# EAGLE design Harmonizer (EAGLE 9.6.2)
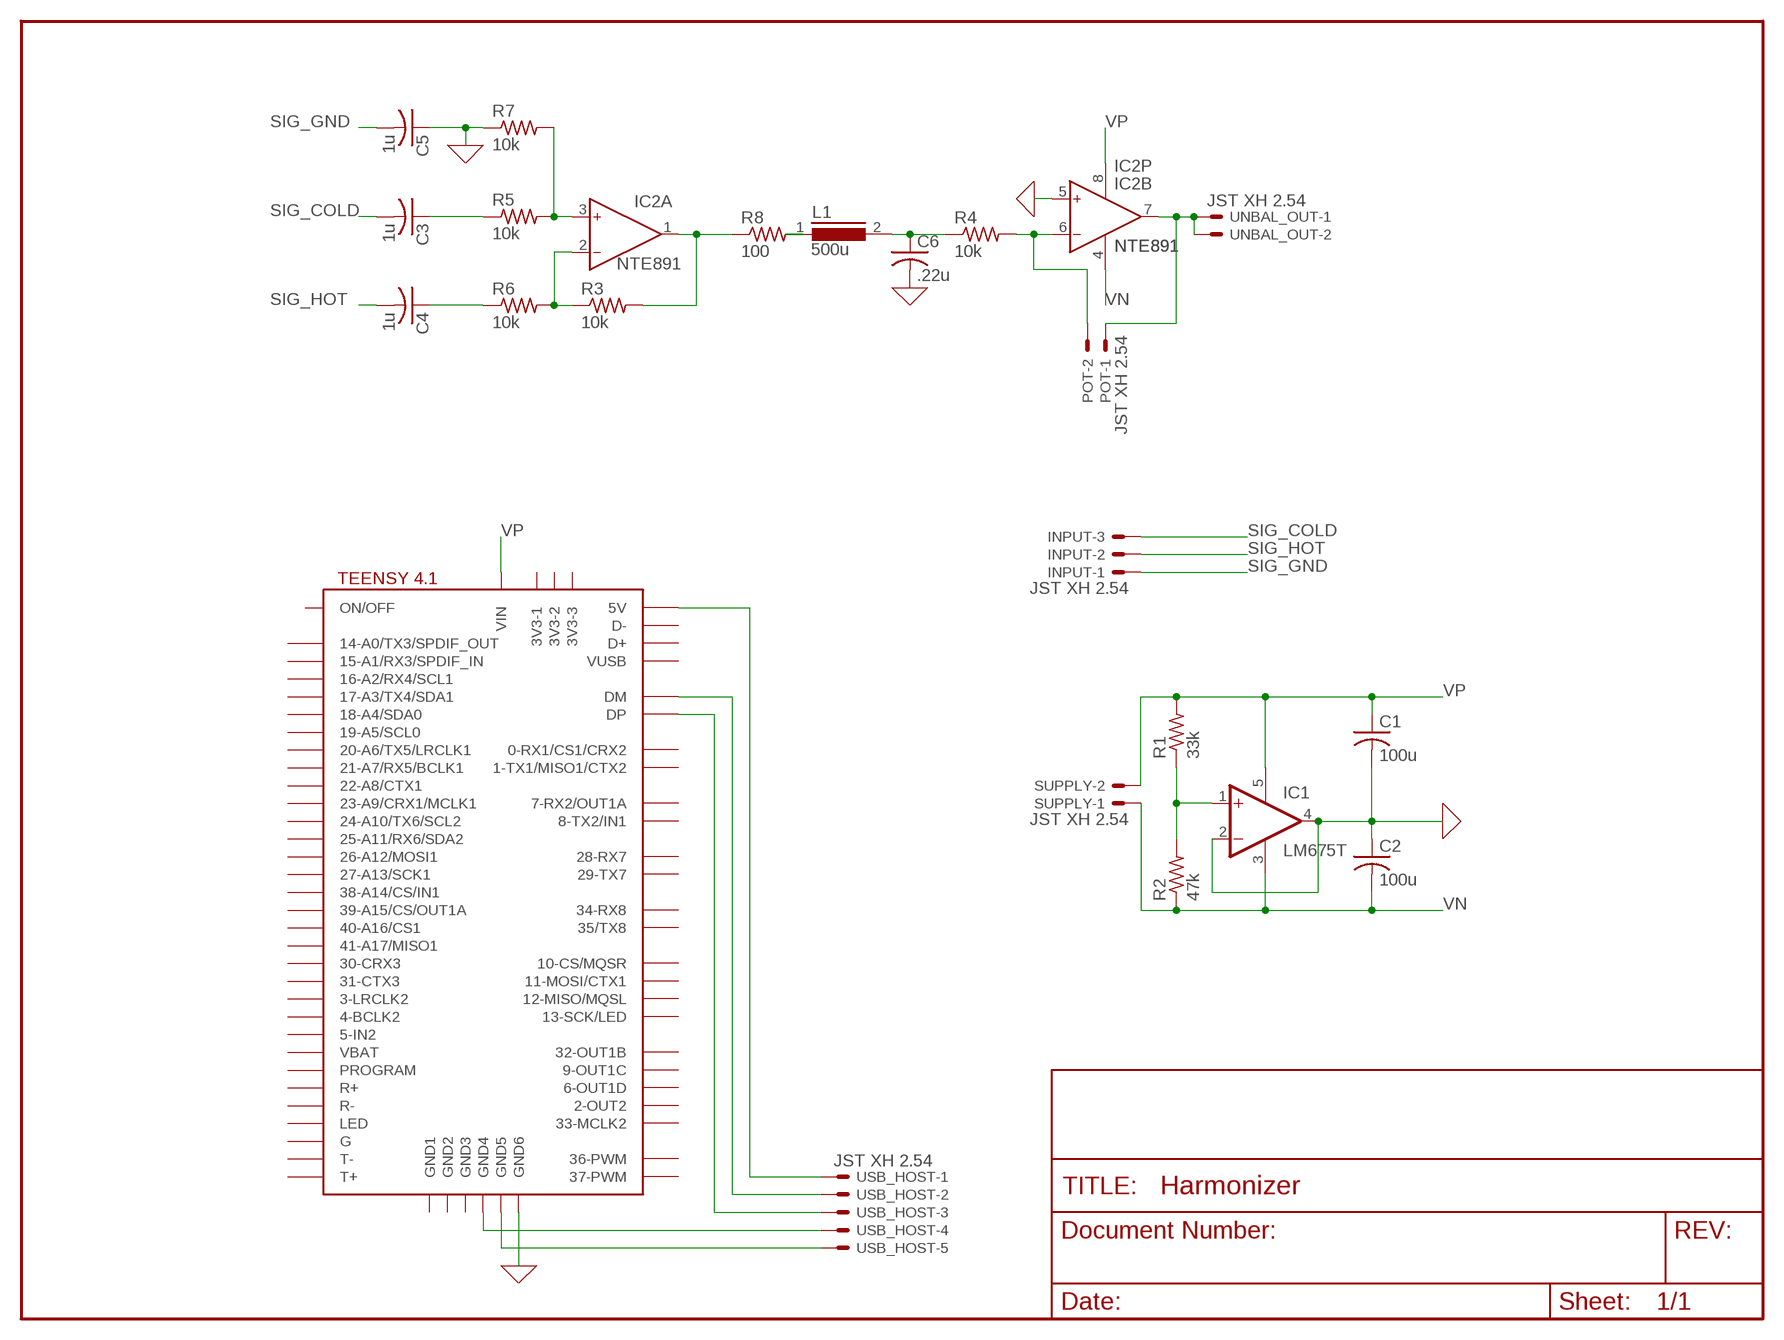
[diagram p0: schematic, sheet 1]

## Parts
C1  100u  C-USC025-050X050-BANTAM  [C025-050X050-BANTAM]
C2  100u  C-USC025-050X050-BANTAM  [C025-050X050-BANTAM]
C3  1u  C-USC025-050X050-BANTAM  [C025-050X050-BANTAM]
C4  1u  C-USC025-050X050-BANTAM  [C025-050X050-BANTAM]
C5  1u  C-USC025-050X050-BANTAM  [C025-050X050-BANTAM]
C6  .22u  C-USC025-050X050-BANTAM  [C025-050X050-BANTAM]
IC1  LM675T  [CB367]
IC2  NTE891  AD822N  [DIL08]
INPUT  JST XH 2.54  22-23-2031  [22-23-2031]
L1  500u  B82134  [SUKW4-32]
POT  JST XH 2.54  22-23-2021  [22-23-2021]
R1  33k  R-US_0207/10-BANTAM  [0207/10-BANTAM]
R2  47k  R-US_0207/10-BANTAM  [0207/10-BANTAM]
R3  10k  R-US_0207/10-BANTAM  [0207/10-BANTAM]
R4  10k  R-US_0207/10-BANTAM  [0207/10-BANTAM]
R5  10k  R-US_0207/10-BANTAM  [0207/10-BANTAM]
R6  10k  R-US_0207/10-BANTAM  [0207/10-BANTAM]
R7  10k  R-US_0207/10-BANTAM  [0207/10-BANTAM]
R8  100  R-US_0207/10-BANTAM  [0207/10-BANTAM]
SUPPLY  JST XH 2.54  22-27-2021-02  [6410-02]
U$1  TEENSY41  [TEENSY41]
UNBAL_OUT  JST XH 2.54  22-27-2021-02  [6410-02]
USB_HOST  JST XH 2.54  22-27-2051-05  [6410-05]

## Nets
0: C1.2 C2.1 C5.1 C6.2 IC1.2(-IN) IC1.4(OUT) IC2.5(B:IN+) R7.1 U$1.GND6 ; supply symbol labelled GND
N$1: IC2.1(A:OUT) R3.2 R8.1
N$2: IC2.6(B:IN-) POT.2 R4.2
N$3: C6.1 L1.2 R4.1
N$4: IC2.2(A:IN-) R3.1 R6.2
N$5: IC2.3(A:IN+) R5.2 R7.2
N$6: L1.1 R8.2
N$7: IC1.1(+IN) R1.1 R2.2
N$8: C3.1 R5.1
N$9: C4.1 R6.1
N$10: U$1.GND5 USB_HOST.5
N$11: U$1.GND4 USB_HOST.4
N$12: U$1.DP USB_HOST.3
N$13: U$1.DM USB_HOST.2
N$14: U$1.+5V(5V) USB_HOST.1
SIG_COLD: C3.2 INPUT.3
SIG_GND: C5.2 INPUT.1
SIG_HOT: C4.2 INPUT.2
UNBAL_OUT: IC2.7(B:OUT) POT.1 UNBAL_OUT.1 UNBAL_OUT.2
VN: C2.2 IC1.3(V-) IC2.4(P:V-) R2.1 SUPPLY.1
VP: C1.1 IC1.5(V+) IC2.8(P:V+) R1.2 SUPPLY.2 U$1.VIN
Unconnected: U$1.0-RX1/CS1/CRX2 U$1.1-TX1/MISO1/CTX2 U$1.2-OUT2 U$1.3-LRCLK2 U$1.3V3-1 U$1.3V3-2 U$1.3V3-3 U$1.4-BCLK2 U$1.5-IN2 U$1.6-OUT1D U$1.7-RX2/OUT1A U$1.8-TX2/IN2(8-TX2/IN1) U$1.9-OUT1C U$1.10-CS\MQSR(10-CS/MQSR) U$1.11-MOSI/CTX1 U$1.12-MISO/MQSL U$1.13-SCK/LED U$1.14-A0/TX3/SPDIF_OUT U$1.15-A1/RX3/SPDIF_IN U$1.16-A2/RX4/SCL1 U$1.17-A3/TX4/SDA1 U$1.18-A4/SDA0 U$1.19-A5/SCL0 U$1.20-A6/TX5/LRCLK1 U$1.21-A7/RX5/BCLK1 U$1.22-A8/CTX1 U$1.23-A9/CRX1/MCLK1 U$1.24-A10/TX6/SCL2 U$1.25-A11/RX6/SDA2 U$1.26-A12/MOSI1 U$1.27-A13/SCK1 U$1.28-RX7 U$1.29-TX7 U$1.30-CRX3 U$1.31-CTX3 U$1.32-OUT1B U$1.33-MCLK2 U$1.34-RX8 U$1.35-TX8(35/TX8) U$1.36-PWM U$1.37-PWM U$1.38-A14/CS/IN1 U$1.39-A15/CS/OUT1A U$1.40-A16/CS1 U$1.41-A17/MISO1 U$1.D+ U$1.D- U$1.G U$1.GND1 U$1.GND2 U$1.GND3 U$1.LED U$1.ON/OFF U$1.PROGRAM U$1.R+ U$1.R- U$1.T+ U$1.T- U$1.VBAT U$1.VUSB

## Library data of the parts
C1-C6 = rcl-custom:C-US: CAPACITOR, American symbol
IC1 = linear:LM675T: Power OP AMP
IC2 = analog-devices:AD822: Single-Supply, Rail-to-Rail Low Power FET-Input Op Amp Source: http://www.analog.com/static/imported-files/data_sheets/AD822.pdf; OC_FARNELL: 1438581; OC_NEWARK: unknown
INPUT = con-molex:22-23-2031: .100" (2.54mm) Center Header - 3 Pin; MF: MOLEX; MPN: 22-23-2031; OC_FARNELL: 1462950; OC_NEWARK: 30C0862
L1 = inductors:B82134: INDUCTOR; SPICEPREFIX: L
POT = con-molex:22-23-2021: .100" (2.54mm) Center Header - 2 Pin; MF: MOLEX; MPN: 22-23-2021; OC_FARNELL: 1462926; OC_NEWARK: 25C3832
R1-R8 = rcl-custom:R-US_: RESISTOR, American symbol
SUPPLY UNBAL_OUT = con-molex:22-?-02: CONNECTOR; MF: MOLEX; OC_FARNELL: unknown; OC_NEWARK: unknown
U$1 = TeensyReducedPinout:TEENSY41
USB_HOST = con-molex:22-?-05: CONNECTOR wire to board 2.54 mm (.1 inch) pitch header; MF: MOLEX; OC_FARNELL: unknown; OC_NEWARK: unknown

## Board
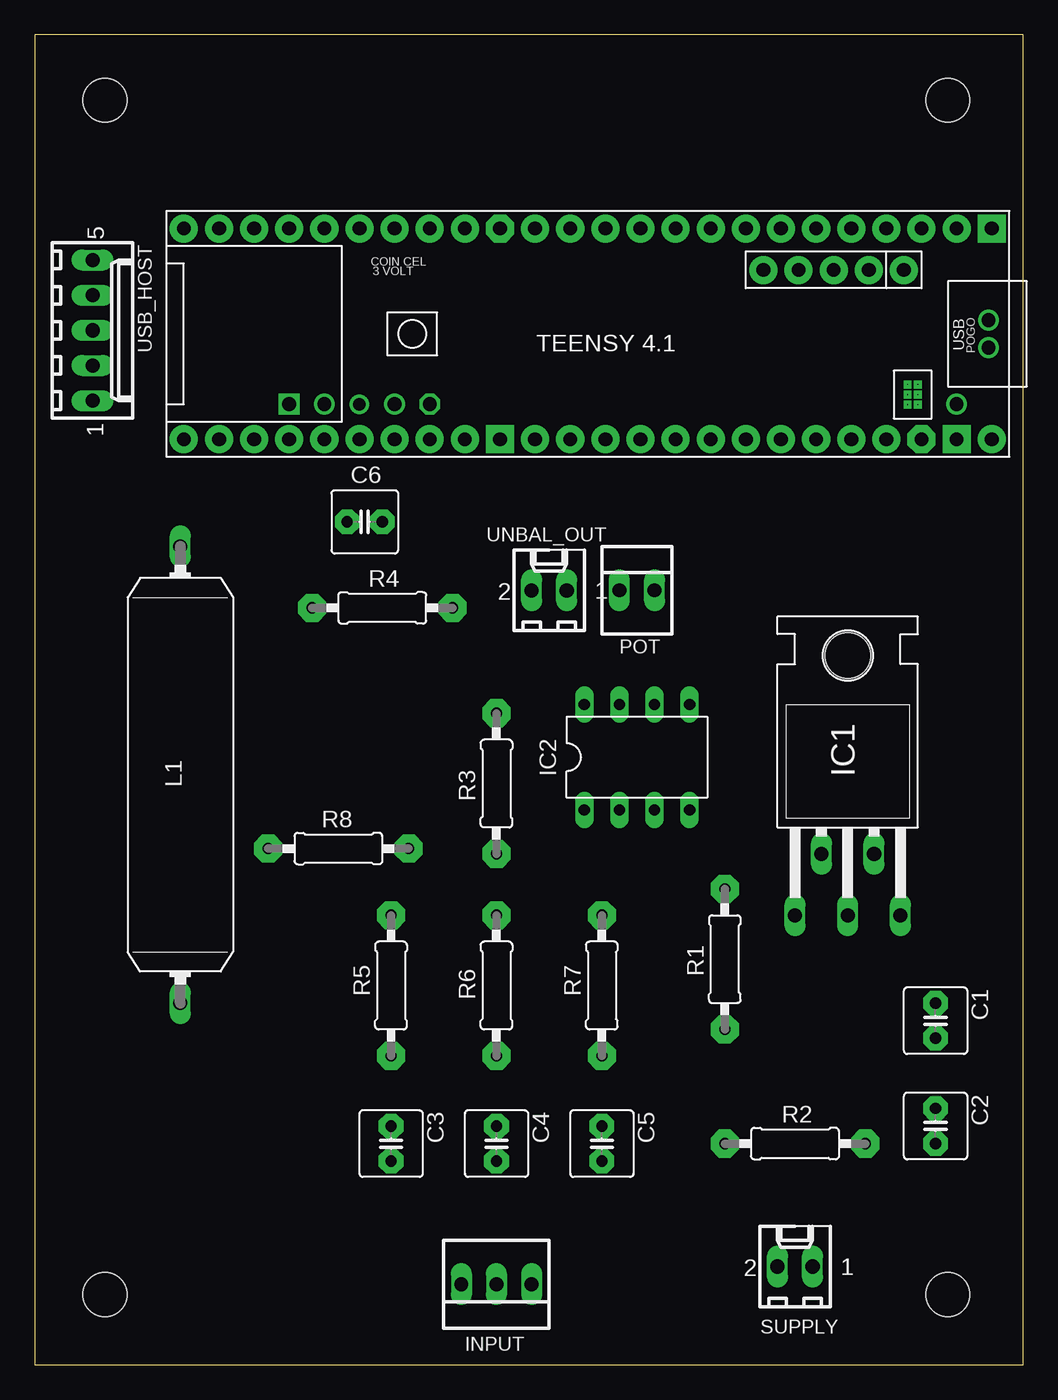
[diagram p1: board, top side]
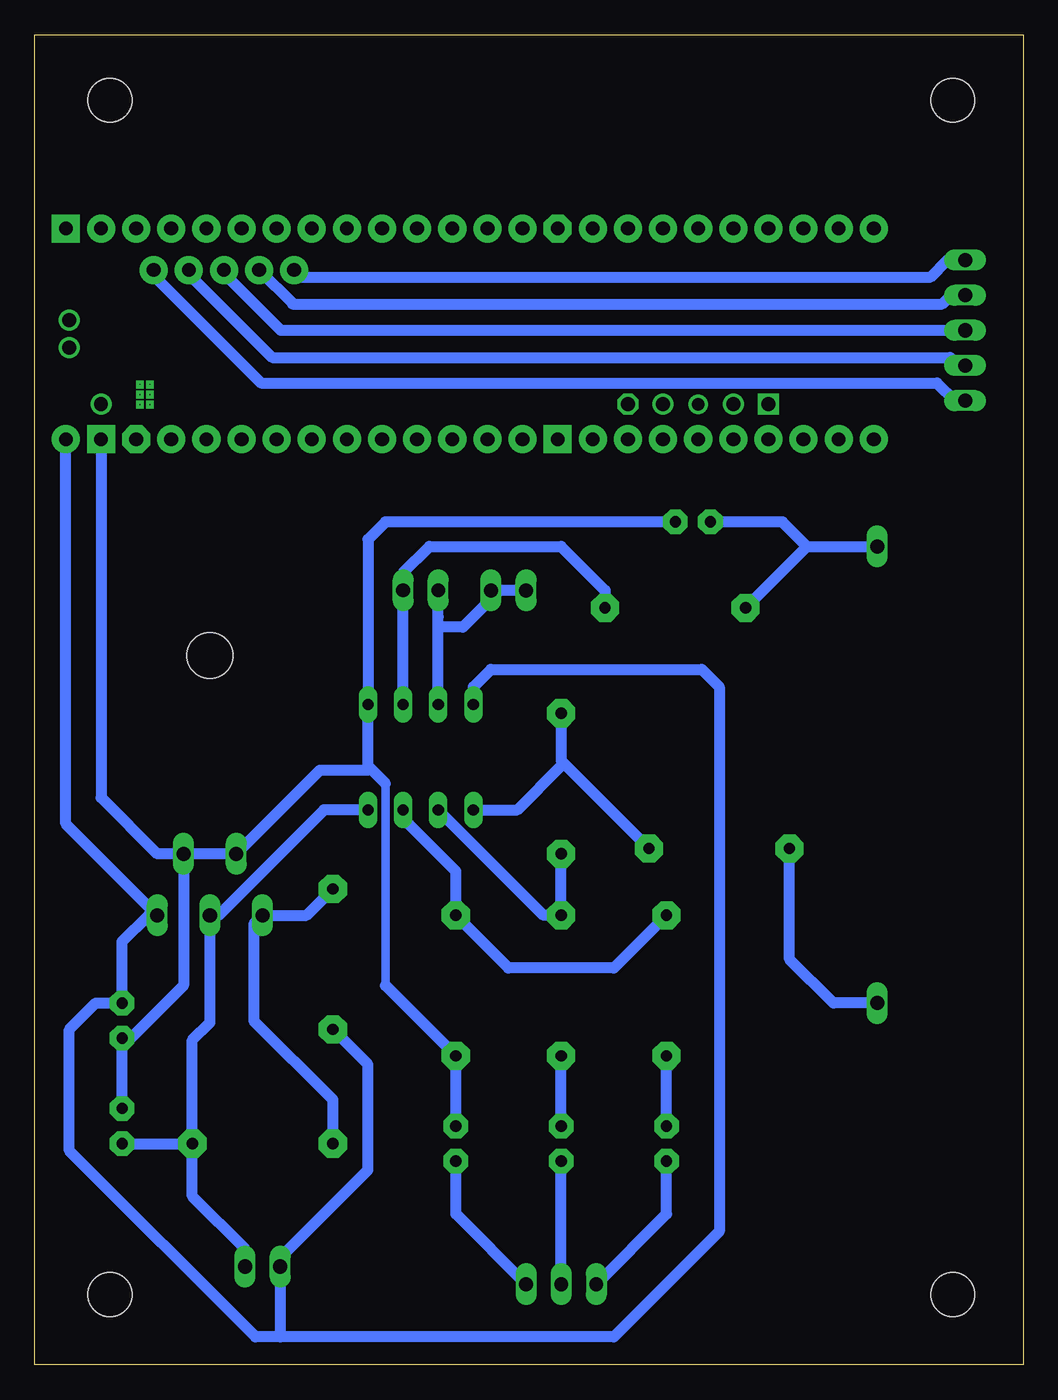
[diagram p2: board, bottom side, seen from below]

Size 71.48 x 96.19 mm. Coordinates in mm from the lower left corner, seen from the top.
Outline: 0,0 71.48,0 71.48,96.19 0,96.19 0,0
Copper layers (1*16): Top 0.035mm / dielectric 1.5mm / Bottom 0.035mm
Design rules "default": minimum track width 6mil, minimum drill 0.35mm, track to track 6mil, track to pad 6mil, pad to pad 6mil, via to via 6mil, smd to smd 6mil, copper to edge 40mil, drill to drill 6mil, minimum pad ring 10mil, minimum via ring 8mil, stop-mask expansion 4mil, vias tented up to drill 0mil, thermal gap 10mil
Holes 3.17 mm at 66.04,5.08 5.08,5.08 5.08,91.44 66.04,91.44

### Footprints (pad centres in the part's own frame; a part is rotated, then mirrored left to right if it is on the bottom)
C025-050X050-BANTAM = drill 0.813 pad 1.778 octagon: 1 -1.27,0; 2 1.27,0
CB367 = drill 1.016 long: 1 -3.81,-11.43; 2 -1.905,-6.985; 3 0,-11.43; 4 1.905,-6.985; 5 3.81,-11.43 | hole 3.302: 0,7.366
DIL08 = drill 0.813 long: 1 -3.81,-3.81; 2 -1.27,-3.81; 3 1.27,-3.81; 4 3.81,-3.81; 5 3.81,3.81; 6 1.27,3.81; 7 -1.27,3.81; 8 -3.81,3.81
22-23-2031 = drill 1 long: 1 -2.54,0; 2 0,0; 3 2.54,0
SUKW4-32 = drill 1.016 long: 1 -16.51,0; 2 16.51,0
22-23-2021 = drill 1 long: 1 -1.27,0; 2 1.27,0
0207/10-BANTAM = drill 0.813 pad 2.032 octagon: 1 -5.08,0; 2 5.08,0
6410-02 = drill 1.016 long: 1 1.27,0; 2 -1.27,0
TEENSY41 = drill 1 pad 2.032: 0-RX1/CS1/CRX2 -27.94,-7.62; 1-TX1/MISO1/CTX2 -25.4,-7.62; 2-OUT2 -22.86,-7.62; 3-LRCLK2 -20.32,-7.62; 4-BCLK2 -17.78,-7.62; 5-IN2 -15.24,-7.62; 6-OUT1D -12.7,-7.62; 7-RX2/OUT1A -10.16,-7.62; 8-TX2/IN2 -7.62,-7.62; 9-OUT1C -5.08,-7.62; 10-CS\MQSR -2.54,-7.62; 11-MOSI/CTX1 0,-7.62; 12-MISO/MQSL 2.54,-7.62; 13-SCK/LED 2.54,7.62; 14-A0/TX3/SPDIF_OUT 0,7.62; 15-A1/RX3/SPDIF_IN -2.54,7.62; 16-A2/RX4/SCL1 -5.08,7.62; 17-A3/TX4/SDA1 -7.62,7.62; 18-A4/SDA0 -10.16,7.62; 19-A5/SCL0 -12.7,7.62; 20-A6/TX5/LRCLK1 -15.24,7.62; 21-A7/RX5/BCLK1 -17.78,7.62; 22-A8/CTX1 -20.32,7.62; 23-A9/CRX1/MCLK1 -22.86,7.62; 24-A10/TX6/SCL2 7.62,-7.62; 25-A11/RX6/SDA2 10.16,-7.62; 26-A12/MOSI1 12.7,-7.62; 27-A13/SCK1 15.24,-7.62; 28-RX7 17.78,-7.62; 29-TX7 20.32,-7.62; 30-CRX3 22.86,-7.62; 31-CTX3 25.4,-7.62; 32-OUT1B 27.94,-7.62; 33-MCLK2 27.94,7.62; 34-RX8 25.4,7.62; 35-TX8 22.86,7.62; 36-PWM 20.32,7.62; 37-PWM 17.78,7.62; 38-A14/CS/IN1 15.24,7.62; 39-A15/CS/OUT1A 12.7,7.62; 40-A16/CS1 10.16,7.62; 41-A17/MISO1 7.62,7.62; +5V -24.13,-4.62; DM -21.59,-4.62; DP -19.05,-4.62; GND4 -16.51,-4.62; GND5 -13.97,-4.62; VIN -30.48,7.62 | drill 1 pad 2.032 octagon: 3V3-1 5.08,-7.62; 3V3-3 -25.4,7.62 | drill 1 pad 0.025: 3V3-2 17.78,5.08; PROGRAM 12.7,5.08 | drill 1: D+ -30.25,-1; D- -30.25,1; VUSB -27.94,5.08 | drill 0.051 pad 0.025 square: G -24.4,4.39; LED -25.13,4.39; R+ -25.13,5.12; R- -24.4,5.12; T+ -24.4,3.66; T- -25.13,3.66 | drill 1 pad 2.032 square: GND1 -30.48,-7.62; GND3 5.08,7.62; GND6 -27.94,7.62 | drill 0.9 pad 0.025: GND2 15.24,5.08 | drill 1 pad 0.025 octagon: ON/OFF 10.16,5.08 | drill 1 pad 0.025 square: VBAT 20.32,5.08
6410-05 = drill 1.016 long: 1 5.08,0; 2 2.54,0; 3 0,0; 4 -2.54,0; 5 -5.08,0

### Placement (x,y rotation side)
C1  65.15,24.89 270 top
C2  65.15,17.27 270 top
C3  25.78,16 270 top
C4  33.4,16 270 top
C5  41.02,16 270 top
C6  23.88,60.96 0 top
IC1  58.8,43.94 0 top
IC2  43.56,43.94 0 top
INPUT  33.4,5.84 180 top
L1  10.54,42.67 90 top
POT  43.56,56.01 0 top
R1  49.91,29.34 270 top
R2  54.99,16 180 top
R3  33.4,42.04 90 top
R4  25.15,54.74 0 top
R5  25.78,27.43 90 top
R6  33.4,27.43 90 top
R7  41.02,27.43 90 top
R8  21.97,37.34 180 top
SUPPLY  54.99,7.11 0 top
U$1  38.73,74.55 180 top
UNBAL_OUT  37.21,56.01 0 top
USB_HOST  4.19,74.8 270 top

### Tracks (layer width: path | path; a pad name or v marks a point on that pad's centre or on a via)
0
  Bottom 0.61: 46.1,42.04 46.1,27.43
  Bottom 0.813: C2.1 C1.2 64.52,23.62 60.71,27.43 IC1.4 | IC1.4 IC1.2 50.86,42.99 47.37,42.99 47.37,43.31 | C5.1 R7.1 46.1,27.43 | IC1.4 62.61,36.96 66.67,41.02 U$1.GND6 | 47.37,43.31 46.1,42.04 | C6.2 46.1,60.96 47.37,59.69 IC2.5 47.37,43.31
N$1
  Bottom 0.61: 33.4,43.31 R3.2
  Bottom 0.813: IC2.1 36.58,40.13 33.4,43.31 | R3.2 33.4,43.69 R8.1
N$2
  Bottom 0.61: POT.2 44.83,57.28
  Bottom 0.813: IC2.6 POT.2 | R4.2 30.23,56.01 33.4,59.18 42.93,59.18 44.83,57.28
N$3
  Bottom 0.813: 15.62,59.18 17.4,60.96 C6.1 | R4.1 15.62,59.18 | 15.62,59.18 L1.2
N$4
  Bottom 0.813: IC2.2 34.67,32.51 R6.2 R3.1
N$5
  Bottom 0.61: 44.83,39.5 IC2.3
  Bottom 0.813: R5.2 29.59,28.7 37.21,28.7 R7.2 41.02,35.69 44.83,39.5
N$6
  Bottom 0.813: L1.1 13.72,26.16 16.89,29.34 R8.2
N$7
  Bottom 0.813: R2.2 49.91,19.18 55.63,24.89 55.63,31.88 IC1.1 51.82,32.51 R1.1
N$8
  Bottom 0.813: C3.1 R5.1
N$9
  Bottom 0.813: C4.1 R6.1
N$10
  Bottom 0.813: U$1.GND5 52.2,78.66 6.68,78.66 5.46,79.88 USB_HOST.5
N$11
  Bottom 0.813: U$1.GND4 52.83,76.76 52.83,76.71 5.84,76.71 5.21,77.34 USB_HOST.4
N$12
  Bottom 0.406: U$1.DP 57.78,78.92
  Bottom 0.813: 57.78,78.92 53.67,74.8 USB_HOST.3
N$13
  Bottom 0.406: 4.7,72.26 USB_HOST.2 | U$1.DM 60.33,78.88
  Bottom 0.813: 4.7,72.26 5.28,72.85 54.29,72.85 60.33,78.88
N$14
  Bottom 0.406: U$1.+5V 62.87,78.75
  Bottom 0.813: USB_HOST.1 4.95,69.72 6.22,71 55.11,71 62.87,78.75
SIG_COLD
  Bottom 0.813: INPUT.3 25.78,10.92 C3.2
SIG_GND
  Bottom 0.813: C5.2 41.02,10.92 INPUT.1
SIG_HOT
  Bottom 0.813: INPUT.2 C4.2
UNBAL_OUT
  Bottom 0.61: 37.85,56.01 UNBAL_OUT.1
  Bottom 0.813: UNBAL_OUT.2 37.85,56.01 40.51,53.34 42.29,53.34 | IC2.7 42.29,53.34 | 42.29,53.34 42.29,54.1 POT.1
VN
  Bottom 0.61: 58.17,32.51 IC1.3
  Bottom 0.813: C2.2 R2.1 | SUPPLY.1 56.26,8.38 60.07,12.19 R2.1 | R2.1 60.07,23.5 58.8,24.77 IC1.3 | IC2.4 50.55,40.13 58.17,32.51
VP
  Bottom 0.61: 63.25,32.51 IC1.5
  Bottom 0.813: 53.72,2.03 SUPPLY.2 53.72,7.75 47.37,14.1 47.37,21.72 R1.2 | 63.25,32.51 65.15,30.61 C1.1 67.06,26.16 68.96,24.26 68.96,15.49 55.5,2.03 53.72,2.03 | IC1.5 69.22,39.12 U$1.VIN | IC2.8 39.75,49.02 38.48,50.29 23.24,50.29 21.97,49.02 21.97,9.65 29.59,2.03 53.72,2.03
